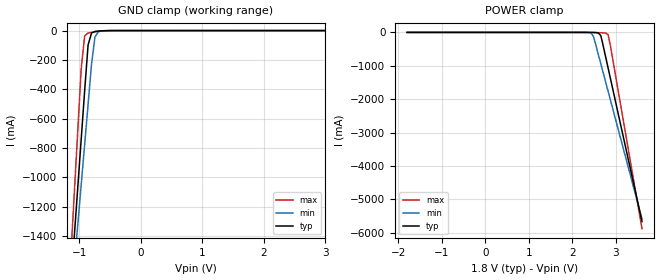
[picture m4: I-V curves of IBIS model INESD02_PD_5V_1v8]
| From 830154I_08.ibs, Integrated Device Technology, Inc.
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[Model] INESD02_PD_5V_1v8
Model_type   Input
Polarity   Non-Inverting
Vinl = 0.630V
Vinh = 1.170V
|   typ   min   max
C_comp   2pF   1.5pF   2.5pF
|   typ   min   max
[Voltage range]  1.8V   1.710V   1.89V
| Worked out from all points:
|   GND clamp passes 1 mA (typ) near -0.59 V on its own axis
[GND_clamp]
|Voltage   I(typ)   I(min)   I(max)
-1.8V     -5.665A    -5.149A    -6.557A
-1.132V   -1.721A    -1.867A    -1.517A
-1.076V   -1.393A    -1.594A    -1.097A
-1.021V   -1.065A    -1.321A    -677.5mA
-964.9mV  -736.3mA   -1.048A    -257.6mA
-909.3mV  -408.2mA   -775.3mA   -35.41mA
-853.6mV  -97.81mA   -502.7mA   -16.38mA
-797.9mV  -16.86mA   -230.3mA   -12.04mA
-742.3mV  -5.785mA   -43.46mA   -8.829mA
-686.6mV  -3.016mA   -8.109mA   -5.958mA
-630.9mV  -1.576mA   -1.783mA   -3.524mA
3.6V      70.14uA    87.7uA     54.35uA
[POWER_clamp]
|Voltage   I(typ)   I(min)   I(max)
-1.8V     70.14uA    85.51uA    55.71uA
2.264V    -86.62uA   -293.7uA   -22.61uA
2.431V    -1.576mA   -22.51mA   -967.9uA
2.487V    -3.016mA   -128.2mA   -2.321mA
2.598V    -16.86mA   -670.7mA   -7.016mA
2.654V    -97.81mA   -943.4mA   -10.02mA
2.765V    -736.3mA   -1.489A    -19.67mA
2.821V    -1.065A    -1.762A    -68.12mA
2.876V    -1.393A    -2.036A    -418.6mA
3.6V      -5.665A    -5.591A    -5.878A
